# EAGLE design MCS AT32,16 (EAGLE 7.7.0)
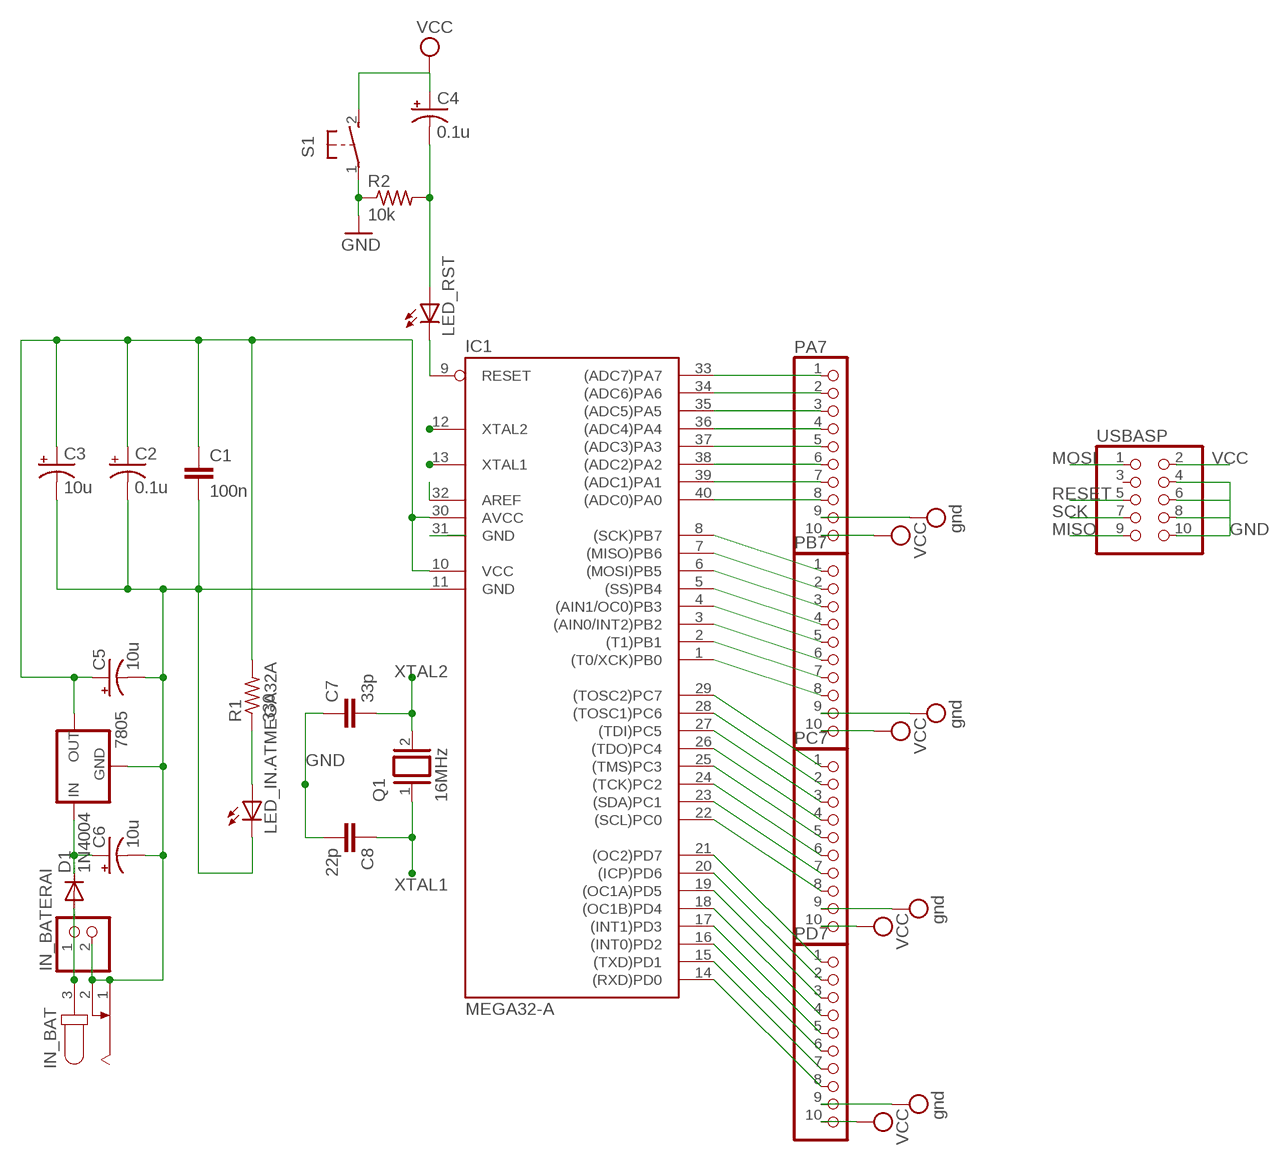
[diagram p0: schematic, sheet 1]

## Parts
7805  78XXL  [78XXL]
C1  100n  C5/3  [C5B3]
C2  0.1u  CPOL-USE1.8-4  [E1,8-4]
C3  10u  CPOL-USE1.8-4  [E1,8-4]
C4  0.1u  CPOL-USE1.8-4  [E1,8-4]
C5  10u  CPOL-USE1.8-4  [E1,8-4]
C6  10u  CPOL-USE1.8-4  [E1,8-4]
C7  33p  C2,5-3  [C2.5-3]
C8  22p  C2,5-3  [C2.5-3]
D1  1N4004  [DO41-10]
IC1  MEGA32-A  MEGA32-P  [DIL40]
IN_BAT  JACK-PLUG0  [SPC4077]
IN_BATERAI  PINHD-1X2/90  [1X02/90]
LED_IN.ATMEGA32A  LED3MM  [LED3MM]
LED_RST  LED3MM  [LED3MM]
PA7  PINHD-1X10  [1X10]
PB7  PINHD-1X10  [1X10]
PC7  PINHD-1X10  [1X10]
PD7  PINHD-1X10  [1X10]
Q1  16MHz  XTAL  [Q]
R1  330  R-US_0207/7  [0207/7]
R2  10k  R-US_0207/7  [0207/7]
S1  31-XX  [B3F-31XX]
USBASP  PINHD-2X5  [2X05]

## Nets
GND: 7805.GND C1.2 C2.- C3.- C5.- C6.- C7.1 C8.2 IC1.11(GND) IC1.31(GND) IN_BAT.1 IN_BAT.2 IN_BATERAI.2 LED_IN.ATMEGA32A.K(C) PA7.9 PB7.9 PC7.9 PD7.9 R2.1 S1.1(P) USBASP.4 USBASP.6 USBASP.8 USBASP.10 ; supply symbol labelled gnd
MISO: IC1.7((MISO)PB6) PB7.2 USBASP.9
MOSI: IC1.6((MOSI)PB5) PB7.3 USBASP.1
N$1: C4.- LED_RST.A R2.2
N$2: IC1.32(AREF)
N$3: D1.A IN_BAT.3 IN_BATERAI.1
N$4: IC1.5((SS)PB4) PB7.4
N$5: IC1.4((AIN1/OC0)PB3) PB7.5
N$6: IC1.3((AIN0/INT2)PB2) PB7.6
N$7: IC1.2((T1)PB1) PB7.7
N$8: IC1.1((T0/XCK)PB0) PB7.8
N$9: IC1.29((TOSC2)PC7) PC7.1
N$10: IC1.28((TOSC1)PC6) PC7.2
N$11: IC1.27((TDI)PC5) PC7.3
N$12: IC1.26((TDO)PC4) PC7.4
N$13: IC1.25((TMS)PC3) PC7.5
N$14: IC1.24((TCK)PC2) PC7.6
N$15: IC1.23((SDA)PC1) PC7.7
N$16: IC1.22((SCL)PC0) PC7.8
N$17: IC1.21((OC2)PD7) PD7.1
N$18: IC1.20((ICP)PD6) PD7.2
N$19: IC1.19((OC1A)PD5) PD7.3
N$20: IC1.18((OC1B)PD4) PD7.4
N$21: IC1.17((INT1)PD3) PD7.5
N$22: IC1.16((INT0)PD2) PD7.6
N$23: IC1.15((TXD)PD1) PD7.7
N$24: IC1.14((RXD)PD0) PD7.8
N$25: IC1.33((ADC7)PA7) PA7.1
N$26: IC1.34((ADC6)PA6) PA7.2
N$27: IC1.35((ADC5)PA5) PA7.3
N$28: IC1.36((ADC4)PA4) PA7.4
N$29: IC1.37((ADC3)PA3) PA7.5
N$30: IC1.38((ADC2)PA2) PA7.6
N$31: IC1.39((ADC1)PA1) PA7.7
N$32: IC1.40((ADC0)PA0) PA7.8
N$33: LED_IN.ATMEGA32A.A R1.1
N$38: 7805.IN C6.+ D1.C
RESET: IC1.9(RESET) LED_RST.K(C) USBASP.5
SCK: IC1.8((SCK)PB7) PB7.1 USBASP.7
VCC: 7805.OUT C1.1 C2.+ C3.+ C4.+ C5.+ IC1.10(VCC) IC1.30(AVCC) PA7.10 PB7.10 PC7.10 PD7.10 R1.2 S1.2(S) USBASP.2
XTAL1: C8.1 IC1.13(XTAL1) Q1.1
XTAL2: C7.2 IC1.12(XTAL2) Q1.2
Unconnected: USBASP.3

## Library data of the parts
7805 = v-reg:78XXL: VOLTAGE REGULATOR
C1 C7 C8 = capacitor-wima:C: CAPACITOR
C2-C6 = rcl:CPOL-US: POLARIZED CAPACITOR, American symbol
D1 = diode:1N4004: DIODE
IC1 = atmel:MEGA32-P: MICROCONTROLLER 32 Kbytes FLASH 2 Kbytes SRAM 1 Kbytes EEPROM USART 8-channel 10 bit ADC Source: www.atmel.com .. doc2503.pdf; MPN: ATMEGA32-16PU; OC_FARNELL: 1661729; OC_NEWARK: 51P1794
IN_BAT = con-jack:JACK-PLUG: DC POWER JACK Power Jack, DC, Right Angle, Through Hole, Rated 5A at 16VDC, PC Terminals Distributor: Farnell (www.Farnell.de) Drawing: 84N1161.pdf / 84N1162.pdf Manufacturer: SPC Technology (www.spctechnology.com) Type: SPC4077 / SPC 4078; OC_FARNELL: unknown; OC_NEWARK: unknown
IN_BATERAI = pinhead:PINHD-1X2: PIN HEADER
LED_IN.ATMEGA32A LED_RST = led:LED: LED
PA7 PB7 PC7 PD7 = pinhead:PINHD-1X10: PIN HEADER
Q1 = special:XTAL: CRYSTAL
R1 R2 = resistor:R-US_: RESISTOR, American symbol
S1 = switch-omron:31-XX: OMRON SWITCH; MPN: B3F-3100; OC_FARNELL: 959704; OC_NEWARK: 36M3582
USBASP = pinhead:PINHD-2X5: PIN HEADER

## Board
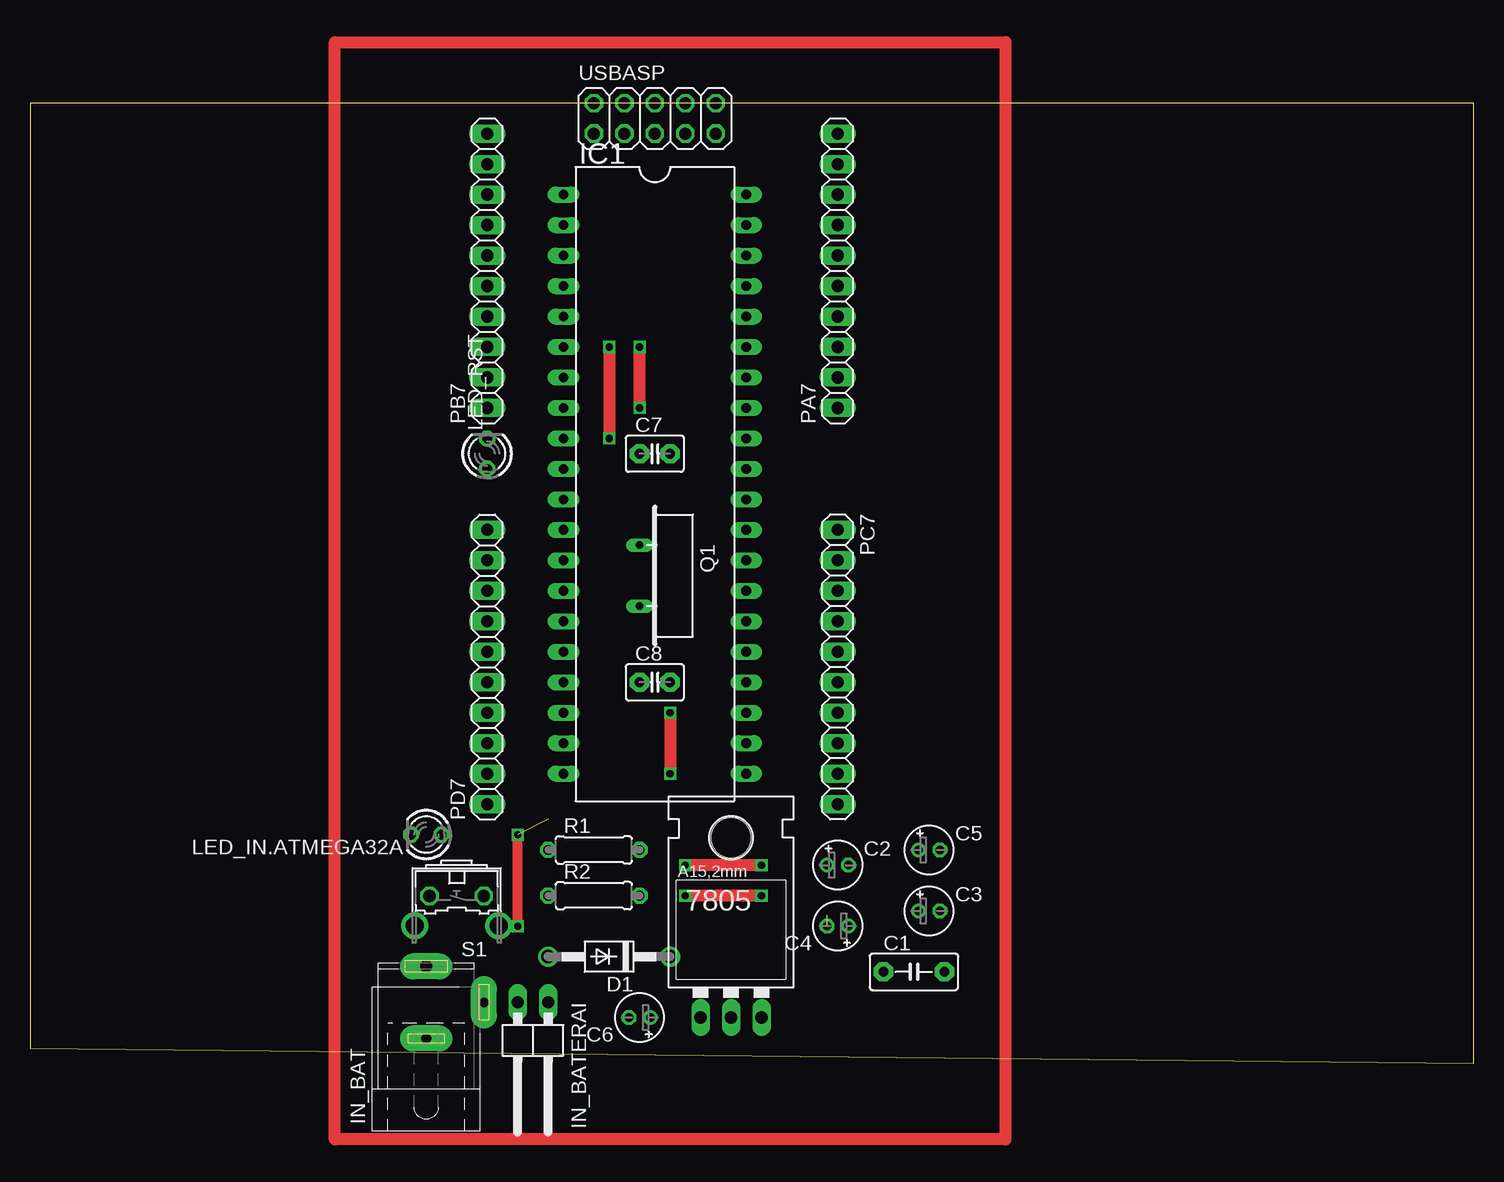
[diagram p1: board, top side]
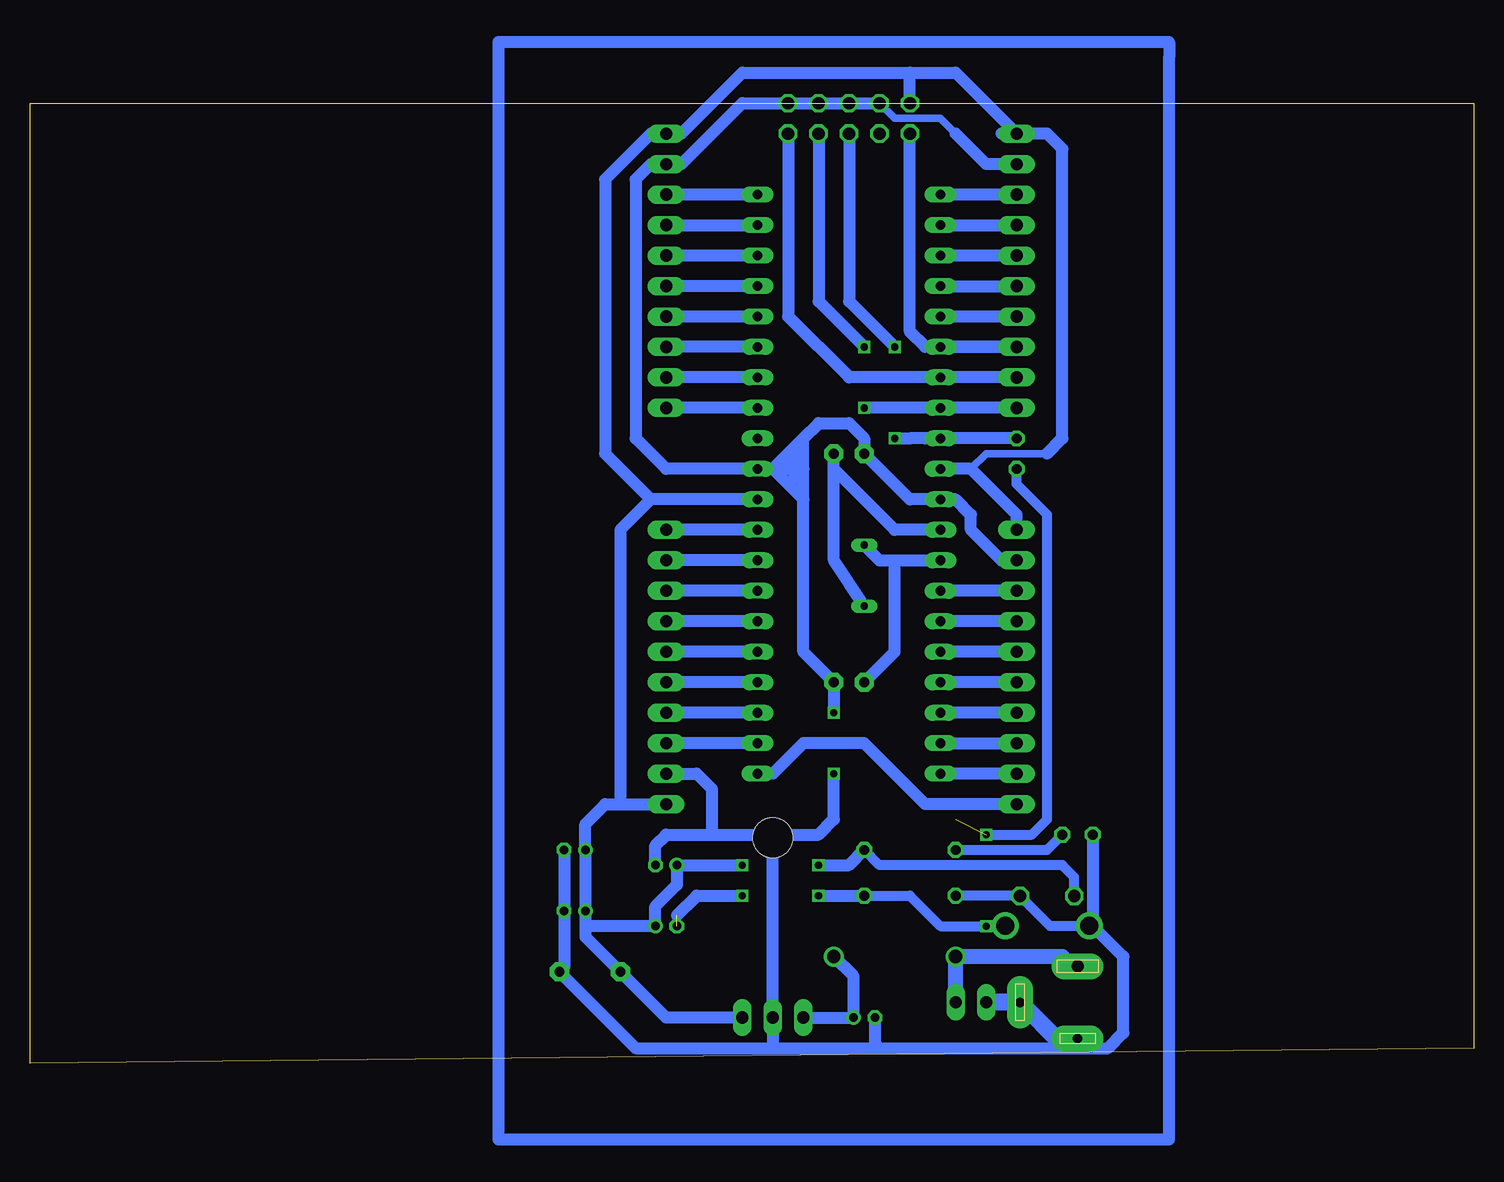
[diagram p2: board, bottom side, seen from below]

Size 120.32 x 80 mm. Coordinates in mm from the lower left corner, seen from the top.
Outline: 0,1.27 120.32,0 120.32,80 0,80 0,1.27
Copper layers (1*16): Top 0.035mm / dielectric 1.5mm / Bottom 0.035mm
Design rules "default": minimum track width 10mil, minimum drill 24mil, track to track 8mil, track to pad 8mil, pad to pad 8mil, via to via 8mil, smd to smd 8mil, copper to edge 40mil, drill to drill 8mil, minimum pad ring 10mil, minimum via ring 8mil, stop-mask expansion 4mil, vias tented up to drill 0mil, thermal gap 10mil

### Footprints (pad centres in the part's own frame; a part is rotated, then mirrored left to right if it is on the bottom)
78XXL = drill 1.016 long: GND 0,-3.81; IN -2.54,-3.81; OUT 2.54,-3.81 | hole 3.302: 0,11.176
C5B3 = drill 0.813 pad 1.6 octagon: 1 -2.54,0; 2 2.54,0
E1,8-4 = drill 0.711 pad 1.168: + -0.889,0 | drill 0.711 pad 1.168 octagon: - 0.889,0
C2.5-3 = drill 0.813 pad 1.6 octagon: 1 -1.27,0; 2 1.27,0
DO41-10 = drill 1.118: A 5.08,0; C -5.08,0
DIL40 = drill 0.813 long: 1 -24.13,-7.62; 2 -21.59,-7.62; 3 -19.05,-7.62; 4 -16.51,-7.62; 5 -13.97,-7.62; 6 -11.43,-7.62; 7 -8.89,-7.62; 8 -6.35,-7.62; 9 -3.81,-7.62; 10 -1.27,-7.62; 11 1.27,-7.62; 12 3.81,-7.62; 13 6.35,-7.62; 14 8.89,-7.62; 15 11.43,-7.62; 16 13.97,-7.62; 17 16.51,-7.62; 18 19.05,-7.62; 19 21.59,-7.62; 20 24.13,-7.62; 21 24.13,7.62; 22 21.59,7.62; 23 19.05,7.62; 24 16.51,7.62; 25 13.97,7.62; 26 11.43,7.62; 27 8.89,7.62; 28 6.35,7.62; 29 3.81,7.62; 30 1.27,7.62; 31 -1.27,7.62; 32 -3.81,7.62; 33 -6.35,7.62; 34 -8.89,7.62; 35 -11.43,7.62; 36 -13.97,7.62; 37 -16.51,7.62; 38 -19.05,7.62; 39 -21.59,7.62; 40 -24.13,7.62
SPC4077 = drill 0.8 pad 2.184 long: 1 -3,0; 2 0,-4.8 | drill 1 pad 2.184 long: 3 3,0
1X02/90 = drill 1.016 long: 1 -1.27,-3.81; 2 1.27,-3.81
LED3MM = drill 0.813 octagon: A -1.27,0; K 1.27,0
1X10 = drill 1.016 long: 1 -11.43,0; 2 -8.89,0; 3 -6.35,0; 4 -3.81,0; 5 -1.27,0; 6 1.27,0; 7 3.81,0; 8 6.35,0; 9 8.89,0; 10 11.43,0
Q = drill 0.61 long: 1 -2.54,-3.81; 2 2.54,-3.81
0207/7 = drill 0.813 octagon: 1 -3.81,0; 2 3.81,0
B3F-31XX = drill 1.016 octagon: 1 -2.261,-1.245; 2 2.261,-1.245 | drill 1.499 pad 2.159: 3 -3.505,1.245; 4 3.505,1.245
2X05 = drill 1.016 octagon: 1 -5.08,-1.27; 2 -5.08,1.27; 3 -2.54,-1.27; 4 -2.54,1.27; 5 0,-1.27; 6 0,1.27; 7 2.54,-1.27; 8 2.54,1.27; 9 5.08,-1.27; 10 5.08,1.27

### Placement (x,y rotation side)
7805  58.42,7.62 0 top
C1  73.66,7.62 0 top
C2  67.31,16.51 0 top
C3  74.93,12.7 0 top
C4  67.31,11.43 180 top
C5  74.93,17.78 0 top
C6  50.8,3.81 180 top
C7  52.07,50.8 0 top
C8  52.07,31.75 0 top
D1  48.26,8.89 180 top
IC1  52.07,48.26 270 top
IN_BAT  33.02,5.08 90 top
IN_BATERAI  41.91,1.27 180 top
LED_IN.ATMEGA32A  33.02,19.05 180 top
LED_RST  38.1,50.8 90 top
PA7  67.31,66.04 90 top
PB7  38.1,66.04 90 top
PC7  67.31,33.02 270 top
PD7  38.1,33.02 90 top
Q1  54.61,40.64 270 top
R1  46.99,17.78 0 top
R2  46.99,13.97 0 top
S1  35.56,12.7 180 top
USBASP  52.07,78.74 0 top

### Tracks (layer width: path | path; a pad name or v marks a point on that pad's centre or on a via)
GND  (via drill 0.6)
  Top 1.016: v53.34,29.21 v53.34,24.13
  Bottom 0.61: 43.18,77.47 44.45,78.74 48.26,78.74 USBASP.4
  Bottom 0.813: 31.75,11.43 35.31,11.43 S1.1 43.16,13.95 | C5.- 75.82,8
  Bottom 1.016: PD7.9 39.37,41.91 41.91,44.45 41.91,45.72 43.18,46.99 IC1.11 46.99,46.99 C7.1 50.8,52.07 52.07,53.34 54.61,53.34 55.88,52.07 | 55.88,46.99 55.88,34.29 C8.2 v53.34,29.21 | 58.42,49.53 IC1.31 67.31,49.53 69.85,52.07 69.85,73.66 68.58,74.93 PA7.9 66.04,74.93 60.96,80.01 USBASP.10 USBASP.8 USBASP.6 USBASP.4 | 58.42,49.53 57.15,48.26 | 57.15,48.26 55.88,46.99 | 55.88,46.99 55.88,49.53 | 55.88,49.53 55.88,52.07 | PB7.9 40.64,74.93 43.18,77.47 | C5.- C3.- 75.82,8 C1.2 69.85,1.27 58.42,1.27 | C2.- 68.2,18.16 67.31,19.05 63.5,19.05 | 63.5,19.05 58.42,19.05 | 58.42,19.05 7805.GND 58.42,1.27 | 55.88,49.53 57.15,49.53 | 57.15,49.53 58.42,49.53 | 57.15,48.26 55.88,49.53 | 58.42,49.53 55.88,52.07 | 55.88,52.07 57.15,49.53 | 58.42,19.05 54.61,19.05 53.34,20.32 v53.34,24.13 | PC7.9 64.77,24.13 63.5,22.86 63.5,19.05 | 49.53,1.27 34.29,1.27 | 34.29,1.27 32.21,1.27 | 32.21,1.27 IN_BAT.1 | C6.- 49.91,1.65 49.53,1.27 | IN_BATERAI.2 38.1,5.08 34.29,1.27 | 32.21,1.27 30.48,1.27 29.21,2.54 29.21,8.89 31.75,11.43 LED_IN.ATMEGA32A.K | 43.16,13.95 R2.1 | 58.42,1.27 49.53,1.27
  Bottom 1.422: IN_BAT.1 34.82,2.08 IN_BAT.2 IN_BATERAI.2
MISO
  Bottom 1.016: PB7.2 IC1.7 52.07,57.15 57.15,62.23 USBASP.9
MOSI
  Bottom 1.016: IC1.6 PB7.3 45.72,59.69 46.99,60.96 USBASP.1
N$1  (via drill 0.6)  (2 unrouted)
  Top 0.813: v40.64,11.43 v40.64,19.05
  Top 1.016: v60.96,13.97 v54.61,13.97
  Bottom 0.813: v40.64,19.05 36.83,19.05 35.56,20.32 35.56,45.72 38.1,48.26 LED_RST.A | R2.2 46.99,13.97 44.45,11.43 v40.64,11.43
  Bottom 1.016: 66.42,12.32 64.77,13.97 v60.96,13.97 | v54.61,13.97 R2.2
N$3
  Bottom 1.27: IN_BATERAI.1 D1.A 34.29,8.89 33.48,8.08 IN_BAT.3
N$4
  Bottom 1.016: PB7.4 IC1.5
N$5
  Bottom 1.016: IC1.4 PB7.5
N$6
  Bottom 1.016: PB7.6 IC1.3
N$7
  Bottom 1.016: IC1.2 PB7.7
N$8
  Bottom 1.016: PB7.8 IC1.1
N$9
  Bottom 1.016: IC1.29 PC7.1
N$10
  Bottom 1.016: IC1.28 PC7.2
N$11
  Bottom 1.016: IC1.27 PC7.3
N$12
  Bottom 1.016: IC1.26 PC7.4
N$13
  Bottom 1.016: IC1.25 PC7.5
N$14
  Bottom 1.016: IC1.24 PC7.6
N$15
  Bottom 1.016: IC1.23 PC7.7
N$16
  Bottom 1.016: IC1.22 PC7.8
N$17
  Bottom 1.016: PD7.1 45.72,21.59 50.8,26.67 55.88,26.67 58.42,24.13 IC1.21
N$18
  Bottom 1.016: PD7.2 IC1.20
N$19
  Bottom 1.016: IC1.19 PD7.3
N$20
  Bottom 1.016: PD7.4 IC1.18
N$21
  Bottom 1.016: PD7.5 IC1.17
N$22
  Bottom 1.016: PD7.6 IC1.16
N$23
  Bottom 1.016: PD7.7 IC1.15
N$24
  Bottom 1.016: PD7.8 IC1.14
N$25
  Bottom 1.016: IC1.33 PA7.1
N$26
  Bottom 1.016: IC1.34 PA7.2
N$27
  Bottom 1.016: IC1.35 PA7.3
N$28
  Bottom 1.016: IC1.36 PA7.4
N$29
  Bottom 1.016: IC1.37 PA7.5
N$30
  Bottom 1.016: IC1.38 PA7.6
N$31
  Bottom 1.016: PA7.7 IC1.39
N$32
  Bottom 1.016: IC1.40 PA7.8
N$33
  Bottom 0.813: R1.1 35.56,17.78 LED_IN.ATMEGA32A.A
N$34
  Bottom 1.016: 25.4,85.09 81.28,85.09 81.28,-6.35 25.4,-6.35 25.4,83.82 25.4,85.09
N$35
  Top 1.016: 25.4,85.09 81.28,85.09 81.28,-6.35 25.4,-6.35 25.4,85.09
N$38
  Bottom 1.016: 7805.IN C6.+ 51.69,7.24 D1.C
RESET  (via drill 0.6)
  Top 1.016: v48.26,59.69 v48.26,52.07
  Bottom 1.016: LED_RST.K IC1.9 45.72,52.07 46.99,52.07 v48.26,52.07 | USBASP.5 52.07,63.5 v48.26,59.69
SCK  (via drill 0.6)
  Top 1.016: v50.8,54.61 v50.8,59.69
  Bottom 1.016: PB7.1 IC1.8 v50.8,54.61 | USBASP.7 54.61,63.5 v50.8,59.69
VCC  (via drill 0.6)
  Top 1.016: v60.96,16.51 v54.61,16.51
  Bottom 0.61: 41.91,49.53 40.64,50.8 35.56,50.8
  Bottom 0.813: S1.2 33.3,15.52 34.29,16.51 49.53,16.51 R1.2
  Bottom 1.016: 71.12,21.59 72.39,21.59 74.04,19.94 C5.+ C3.+ 74.04,11.43 | 71.12,21.59 PC7.10 | 74.04,11.43 74.04,10.54 C1.1 67.31,3.81 7805.OUT | 68.58,46.99 71.12,44.45 71.12,21.59 | IC1.30 68.58,46.99 | 68.58,46.99 72.39,50.8 72.39,73.66 68.58,77.47 PA7.10 66.04,77.47 60.96,82.55 46.99,82.55 | 46.99,82.55 43.18,82.55 PB7.10 | USBASP.2 46.99,82.55 | PD7.10 38.1,45.72 41.91,49.53 IC1.10 | v60.96,16.51 C2.+ 66.42,14.86 68.2,13.08 C4.+ 74.04,11.43 | v54.61,16.51 52.07,16.51 R1.2 | 35.56,50.8 34.29,52.07 34.29,76.2 35.56,77.47 PB7.10 | 39.37,77.47 PB7.10
XTAL1
  Bottom 1.016: Q1.1 49.53,41.91 48.26,41.91 | 48.26,41.91 IC1.13 | C8.1 48.26,34.29 48.26,41.91
XTAL2
  Bottom 1.016: Q1.2 53.34,41.91 53.34,49.53 | 53.34,49.53 C7.2 | IC1.12 48.26,44.45 53.34,49.53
